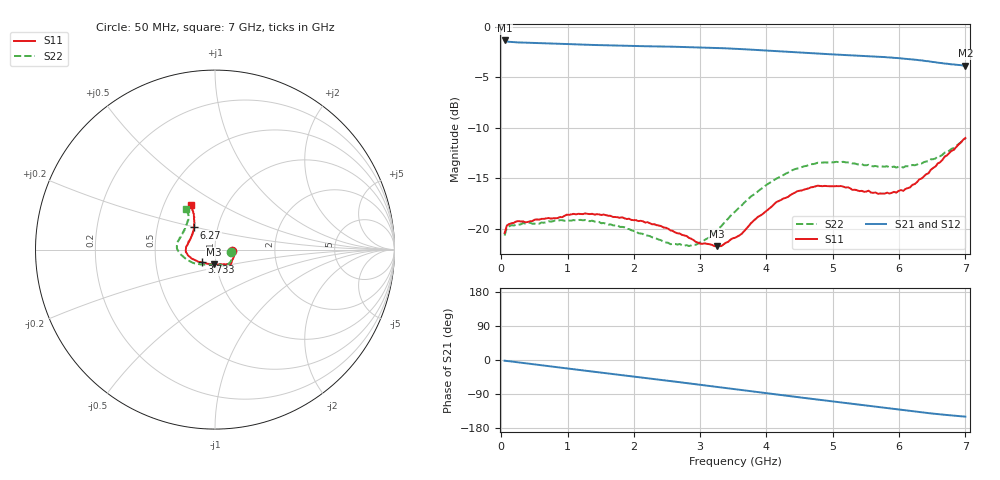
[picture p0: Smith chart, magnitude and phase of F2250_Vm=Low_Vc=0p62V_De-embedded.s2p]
! Integrated Device Technology
! Corporate Headquarters
! 6024 Silver Creek Valley Road
! San Jose, CA 95138  USA
! Phone:  1-408-284-8200
! Toll Free:  1-800-223-1366
! Webpage:  http://www.idt.com/
! Timing and RF Division
! 515 Groton Road, Suite 102
! Westford, MA 01886-6024
! Device:  F2250
! Description: Voltage Variable RF Attenuator
! Frequency:  50.0 -  6000.00 MHz
! Package:  3x3 mm Thin QFN Plastic Package: 16 pin
! Ports:  2 RF, 3 DC
!  Pin  1  = GND
!  Pin  2  = NC
!  Pin  3  = RF1  = Port 1
!  Pin  4  = NC
!  Pin  5  = GND
!  Pin  6  = GND
!  Pin  7  = GND
!  Pin  8  = GND
!  Pin  9  = NC
!  Pin 10  = RF2  = Port 2
!  Pin 11  = NC
!  Pin 12  = GND
!  Pin 13  = GND
!  Pin 14  = VCNTRL
!  Pin 15  = VDD
!  Pin 16  = VMODE
! Vcntrl:  0.620 Volts
! Vmode:  +0.000 Volts
! Vdd:  +3.30  Volts
! Current:  1.141 mA
! Data:  The device was measured on a the F2250 evaluation board which has
!  individual transmission lines to the RF pins.  Data was collected
!  using a calibrated network analyzer.  The evaluation board was
!  de-embedded using a TRL calibration technique.
!  The reference plane is the edge of the package pin.
! Misc:  SN 10
!  Action Tracker AT0258
! Date Measured:  2014-11-26
! Date:  2015-10-15  MJV
! Note:
!  Integrated Device Technology supplies this data as a sample of measured
!  data at the package pin for this product.  Your particular data for this
!  product may vary.
!  Data was taken at 25 degrees C.
!  Integrated Device Technology reserves the right to change this data at anytime.
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# GHz S dB R 50
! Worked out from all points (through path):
!   201 points, 50 MHz to 7 GHz, reference 50 ohm
!   highest |S21| = -1.32 dB at 50 MHz (marker M1); lowest = -3.8 dB at 7 GHz (marker M2)
!   group delay of S21, straight-line fit = 60 ps
!   lowest |S11| = -21.7 dB at 3.247 GHz (marker M3), VSWR 1.18, Z = 48.6 - j7.98 ohm
!   |S11| at or under -10 dB: start of sweep to end of sweep
!   |S22| runs from -21.7 to -11.1 dB; largest |S21 - S12| = 0.0005
!   S11 on the Smith chart (normalised r, x): 50 MHz: 1.21, -0.02; 3.733 GHz: 0.85, -0.12; 6.27 GHz: 0.77, +0.20; 7 GHz: 0.68, +0.37
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0.05  -20.44 -5.6  -1.32 -1.8  -1.32 -1.8  -20.68 -6.8
0.08475  -19.68 -5.8  -1.42 -2.5  -1.42 -2.5  -19.90 -6.6
0.15425  -19.47 -7.9  -1.48 -4.0  -1.48 -4.0  -19.67 -8.5
0.6755  -18.99 -26.3  -1.61 -15.5  -1.61 -15.5  -19.38 -30.4
1.2315  -18.56 -42.8  -1.73 -27.5  -1.73 -27.5  -19.17 -51.6
1.75275  -18.87 -49.7  -1.83 -38.5  -1.83 -38.5  -19.67 -61.9
2.37825  -19.69 -52.8  -1.92 -51.8  -1.92 -51.8  -21.09 -71.6
2.552  -20.18 -55.9  -1.94 -55.6  -1.94 -55.6  -21.55 -77.6
2.83  -20.91 -65.4  -1.99 -61.7  -1.98 -61.7  -21.73 -92.4
3.0385  -21.49 -78.6  -2.02 -66.3  -2.02 -66.3  -21.28 -106.9
3.247  -21.74 -95.0  -2.07 -70.9  -2.07 -70.9  -20.21 -121.3
3.525  -20.91 -120.2  -2.15 -77.1  -2.15 -77.2  -18.33 -138.2
3.7335  -19.73 -136.8  -2.22 -81.8  -2.22 -81.8  -17.01 -148.0
4.1505  -17.36 -157.0  -2.39 -91.0  -2.39 -91.0  -15.03 -165.6
4.46325  -16.30 -167.2  -2.51 -97.8  -2.51 -97.8  -14.03 -174.5
4.7065  -15.87 -174.1  -2.60 -103.0  -2.60 -103.0  -13.59 179.8
5.15825  -15.83 174.8  -2.77 -112.7  -2.77 -112.7  -13.37 169.9
5.85325  -16.51 150.6  -3.01 -127.6  -3.01 -127.6  -13.91 153.8
6.06175  -16.25 142.2  -3.12 -132.1  -3.12 -132.1  -13.94 147.8
6.27025  -15.38 133.5  -3.25 -136.6  -3.25 -136.6  -13.64 141.2
6.61775  -13.41 122.6  -3.55 -143.3  -3.55 -143.4  -12.81 129.5
7  -11.00 118.6  -3.82 -149.5  -3.82 -149.6  -11.07 125.1
